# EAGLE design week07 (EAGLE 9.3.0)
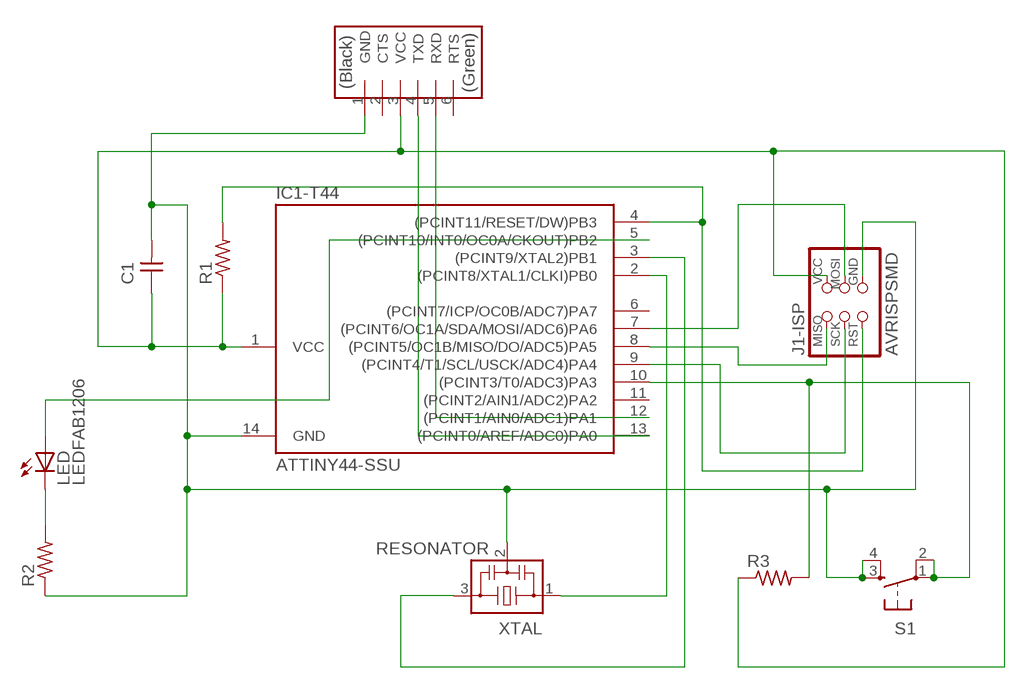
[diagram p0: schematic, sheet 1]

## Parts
C1  CAP-UNPOLARIZEDFAB  [C1206FAB]
IC1-T44  ATTINY44-SSU  [SOIC14]
J1-ISP  AVRISPSMD  [2X03SMD]
J2-FTDI  FTDI-SMD-HEADER  [1X06SMD]
LED  LEDFAB1206  [LED1206FAB]
R1  RES-US1206FAB  [R1206FAB]
R2  RES-US1206FAB  [R1206FAB]
R3  RES-US1206FAB  [R1206FAB]
S1  6MM_SWITCH6MM_SWITCH  [6MM_SWITCH]
XTAL  RESONATOR  [EFOBM]

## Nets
N$1: IC1-T44.7((PCINT6/OC1A/SDA/MOSI/ADC6)PA6) J1-ISP.4(MOSI)
N$2: IC1-T44.8((PCINT5/OC1B/MISO/DO/ADC5)PA5) J1-ISP.1(MISO)
N$3: IC1-T44.9((PCINT4/T1/SCL/USCK/ADC4)PA4) J1-ISP.3(SCK)
N$4: IC1-T44.3((PCINT9/XTAL2)PB1) XTAL.3
N$6: IC1-T44.4((PCINT11/RESET/DW)PB3) J1-ISP.5(RST) R1.2
N$7: IC1-T44.12((PCINT1/AIN0/ADC1)PA1) J2-FTDI.5(RXD)
N$8: IC1-T44.13((PCINT0/AREF/ADC0)PA0) J2-FTDI.4(TXD)
N$9: IC1-T44.2((PCINT8/XTAL1/CLKI)PB0) XTAL.1
N$10: C1.1 IC1-T44.1(VCC) J1-ISP.2(VCC) J2-FTDI.3(VCC) R1.1 R3.1
N$11: LED.2(C) R2.2
N$12: IC1-T44.5((PCINT10/INT0/OC0A/CKOUT)PB2) LED.1(A)
N$13: IC1-T44.10((PCINT3/T0/ADC3)PA3) R3.2 S1.1(P) S1.2(P1)
N$14: C1.2 IC1-T44.14(GND) J1-ISP.6(GND) J2-FTDI.1(GND) R2.1 S1.3(S) S1.4(S1) XTAL.2
Unconnected: IC1-T44.6((PCINT7/ICP/OC0B/ADC7)PA7) IC1-T44.11((PCINT2/AIN1/ADC2)PA2) J2-FTDI.2(CTS) J2-FTDI.6(RTS)

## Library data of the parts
C1 = eagle_fab:CAP-UNPOLARIZED
IC1-T44 = eagle_fab:ATTINY44
J1-ISP = eagle_fab:AVRISP
J2-FTDI = eagle_fab:FTDI-SMD-HEADER
LED = eagle_fab:LED: LED
R1-R3 = eagle_fab:RES-US: Resistor (US Symbol)
S1 = eagle_fab:6MM_SWITCH: OMRON SWITCH
XTAL = eagle_fab:RESONATOR

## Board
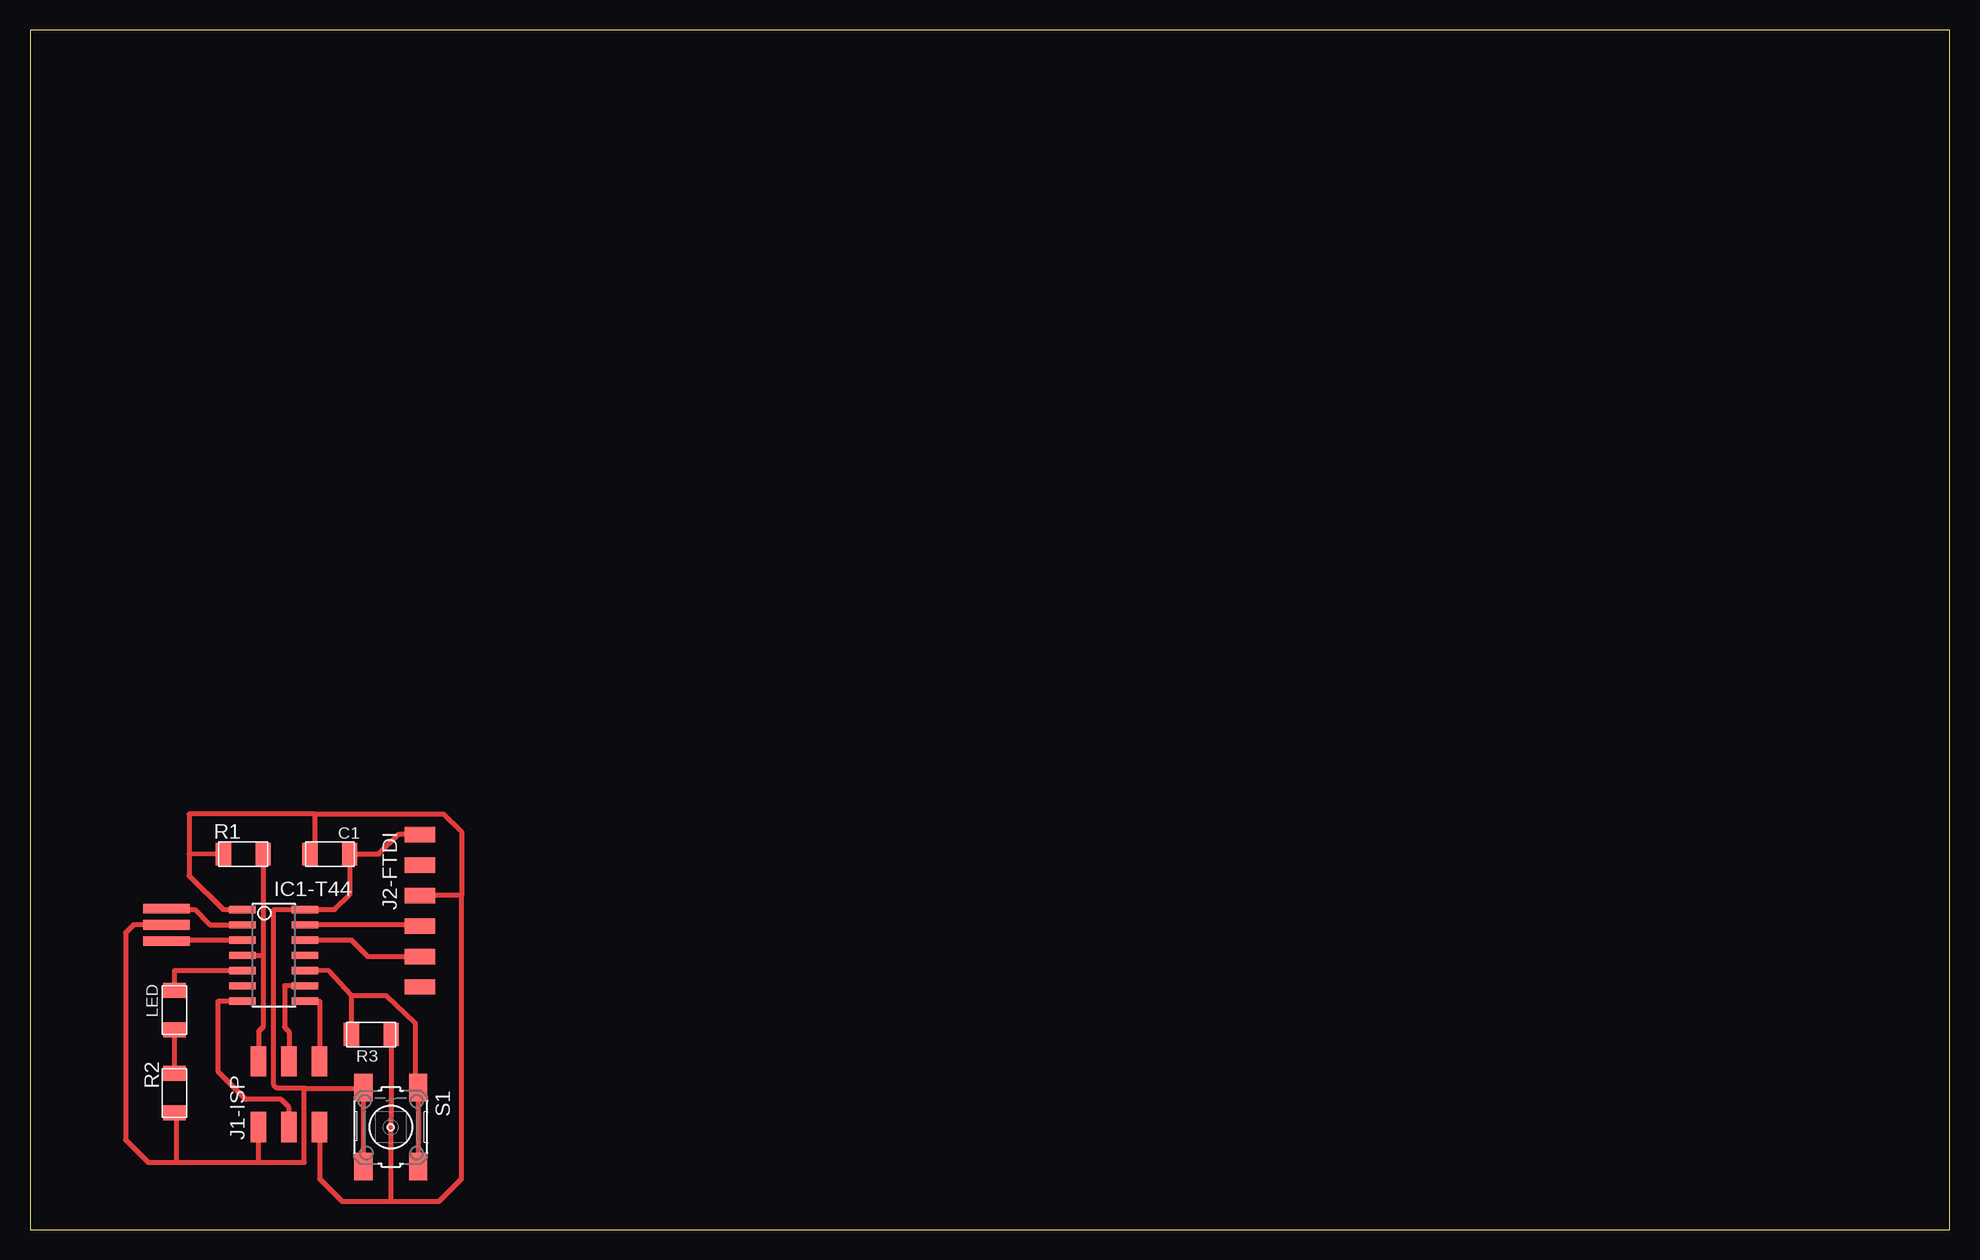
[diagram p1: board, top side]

Size 160 x 100 mm. Coordinates in mm from the lower left corner, seen from the top.
Outline: 0,0 160,0 160,100 0,100 0,0
Copper layers (1*16): Top 0.035mm / dielectric 1.5mm / Bottom 0.035mm
Design rules "eagle_fabcity-designrules *": minimum track width 16mil, minimum drill 32mil, track to track 16mil, track to pad 16mil, pad to pad 16mil, via to via 16mil, smd to smd 16mil, copper to edge 16mil, drill to drill 16mil, minimum pad ring 10mil, minimum via ring 8mil, stop-mask expansion 4mil, vias tented up to drill 0mil, thermal gap 16mil

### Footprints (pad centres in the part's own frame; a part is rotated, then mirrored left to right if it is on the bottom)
C1206FAB = smd 1.27 x 1.905: 1 -1.651,0; 2 1.651,0
SOIC14 = smd 0.61 x 2.21: 1 -3.81,-2.603; 2 -2.54,-2.603; 3 -1.27,-2.603; 4 0,-2.603; 5 1.27,-2.603; 6 2.54,-2.603; 7 3.81,-2.603; 8 3.81,2.603; 9 2.54,2.603; 10 1.27,2.603; 11 0,2.603; 12 -1.27,2.603; 13 -2.54,2.603; 14 -3.81,2.603
2X03SMD = smd 2.54 x 1.27: 1 -2.54,2.54; 2 2.92,2.54; 3 -2.54,0; 4 2.92,0; 5 -2.54,-2.54; 6 2.92,-2.54
1X06SMD = smd 2.54 x 1.27: 1 0,6.35; 2 0,3.81; 3 0,1.27; 4 0,-1.27; 5 0,-3.81; 6 0,-6.35
LED1206FAB = smd 1.27 x 1.905: 1 -1.651,0; 2 1.651,0
R1206FAB = smd 1.27 x 1.905: 1 -1.651,0; 2 1.651,0
6MM_SWITCH = smd 2.286 x 1.524: 1 -3.302,2.286; 2 3.302,2.286; 3 -3.302,-2.286; 4 3.302,-2.286
EFOBM = smd 0.8 x 3.9: 1 -1.35,0; 2 0,0; 3 1.35,0

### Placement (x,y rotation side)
C1  24.99,31.29 0 top
IC1-T44  20.32,22.86 270 top
J1-ISP  21.59,11.48 270 top
J2-FTDI  32.51,26.57 0 top
LED  12.04,18.29 270 top
R1  17.78,31.29 0 top
R2  12.04,11.38 90 top
R3  28.45,16.26 180 top
S1  30.07,8.53 270 top
XTAL  11.38,25.4 270 top

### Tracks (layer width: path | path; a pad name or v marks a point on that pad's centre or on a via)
N$1
  Top 0.406: J1-ISP.4 21.59,10.19 20.93,10.85 17.98,10.85 15.7,13.13 15.7,19.05 IC1-T44.7
N$2
  Top 0.406: IC1-T44.8 24.13,19.05 J1-ISP.1
N$3
  Top 0.406: IC1-T44.9 21.21,20.32 21.21,16.87 21.59,16.49 J1-ISP.3
N$4
  Top 0.406: XTAL.3 11.46,24.13 IC1-T44.3
N$6
  Top 0.406: R1.2 19.43,22.86 | IC1-T44.4 19.43,22.86 | 19.43,22.86 19.43,16.89 19.05,16.51 J1-ISP.5
N$7
  Top 0.406: IC1-T44.12 26.77,24.13 28.14,22.76 J2-FTDI.5
N$8
  Top 0.406: J2-FTDI.4 32.41,25.4 IC1-T44.13
N$9
  Top 0.406: XTAL.1 11.46,26.67 13.72,26.67 14.99,25.4 IC1-T44.2
N$10
  Top 0.406: 23.72,34.65 13.26,34.65 13.26,31.29 | 35.97,27.84 35.97,33.17 34.49,34.65 23.72,34.65 | 35.97,27.84 J2-FTDI.3 | 23.72,34.65 23.72,31.67 C1.1 | J1-ISP.2 24.13,4.22 26.01,2.34 30.07,2.34 | 30.07,2.34 34.09,2.34 35.97,4.22 35.97,27.84 | R3.1 30.07,2.34 | R1.1 13.31,31.29 13.26,31.29 | 13.26,31.29 13.26,29.5 16.09,26.67 IC1-T44.1
N$11
  Top 0.406: LED.2 R2.2
N$12
  Top 0.406: IC1-T44.5 12.04,21.59 LED.1
N$13
  Top 0.406: IC1-T44.10 24.94,21.55 26.82,19.51 | S1.1 32.36,11.38 | 32.36,11.38 S1.2 | 32.36,11.38 32.11,11.63 32.11,17.22 29.67,19.51 26.82,19.51 | R3.2 26.82,19.51
N$14
  Top 0.406: J2-FTDI.1 30.71,32.92 29.08,31.29 C1.2 26.64,27.91 25.4,26.67 IC1-T44.14 20.32,26.67 20.32,12.04 20.57,11.79 22.86,11.79 | XTAL.2 8.64,25.4 7.98,24.74 7.98,7.47 9.86,5.59 12.19,5.59 | 12.19,5.59 19.05,5.59 | 19.05,5.59 J1-ISP.6 | 19.05,5.59 22.86,5.59 22.86,11.79 | R2.1 12.19,9.8 12.19,5.59 | S1.3 27.79,11.79 | 27.79,11.79 S1.4 | 22.86,11.79 27.79,11.79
